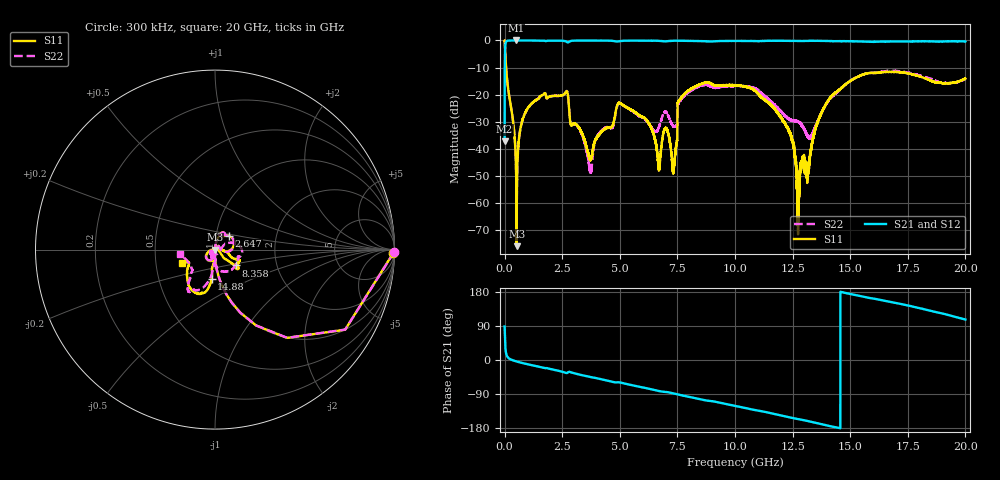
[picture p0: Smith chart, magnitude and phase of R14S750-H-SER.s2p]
!{R14S750}
!Johanson Technology Inc.
!www.johansontechnology.com
!Test Board Conditions:
!Substrate Type  RO4350B
!Substrate Thickness  20 mil
!Substrate Dk  3.66
!TL Type: GCPW
!TL Trace Width  36 mil
!TL Gap  12 mil
!Electrode orientation  Horizontal
!DUT TOPOLOGY	SERIES
!Mounting Pad LxW  26x36 mil
! Created Wed Nov 25 17:33:21 2020
! 2 Port Network Data from SP1.SP block
! freq  magS11  angS11  magS21  angS21  magS12  angS12  magS22  angS22
# khz S ma R 50
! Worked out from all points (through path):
!   20001 points, 300 kHz to 20 GHz, reference 50 ohm
!   highest |S21| = 0.00 dB at 498.3 MHz (marker M1); lowest = -37.2 dB at 300 kHz (marker M2)
!   group delay of S21, straight-line fit = 35 ps
!   lowest |S11| = -75.9 dB at 524.3 MHz (marker M3), VSWR 1.00, Z = 50 - j0.00839 ohm
!   |S11| at or under -10 dB: 64.05 MHz to end of sweep
!   |S22| runs from -70.4 to 0.0 dB; largest |S21 - S12| = 0.017
!   S11 on the Smith chart (normalised r, x): 300 kHz: open; 2.647 GHz: 1.16, +0.18; 8.358 GHz: 1.24, -0.23; 14.88 GHz: 0.91, -0.31; 20 GHz: 0.68, -0.10
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300  0.9937 -1.1  0.01383 88.4  0.01379 89.1  0.9972 -0.9
109300  0.1871 -80.1  0.982 9.9  0.9818 9.9  0.1877 -80.1
498300  0.004191 -92.3  1 -3.6  0.9994 -3.5  0.004227 -95.8
524300  0.0001607 -31.4  0.9993 -4.0  0.9998 -4.0  0.0003109 -154.3
1047300  0.05956 77.4  0.9975 -11.8  0.9976 -11.8  0.05937 78.6
2647300  0.1099 43.8  0.9671 -33.8  0.9674 -33.8  0.1104 42.2
3334300  0.02031 44.5  0.9958 -39.6  0.9965 -39.7  0.0194 41.0
3729300  0.006442 -10.8  0.9934 -45.0  0.9941 -45.0  0.003877 -12.6
5030300  0.0693 -130.6  0.9749 -59.6  0.9745 -59.6  0.06833 -133.7
6226300  0.03073 -168.8  0.9908 -75.3  0.9912 -75.4  0.03037 -142.0
6667300  0.005541 -157.4  0.985 -81.5  0.9846 -81.5  0.02331 -86.2
6999300  0.02413 -114.1  0.9639 -84.4  0.9636 -84.4  0.04792 -95.4
7344300  0.00448 80.8  0.9866 -88.4  0.9881 -88.4  0.02557 -82.8
7600300  0.0806 -41.3  0.9873 -92.0  0.9876 -91.9  0.07508 28.3
8358300  0.1472 -37.0  0.9787 -101.8  0.978 -101.8  0.1378 8.7
1.00003e7  0.1497 -23.8  0.98 -121.1  0.98 -121.1  0.1449 -43.1
1.22063e7  0.02737 3.6  0.9855 -149.2  0.9876 -149.1  0.0389 -123.2
1.27423e7  0.0004717 155.2  0.9756 -156.0  0.9773 -156.1  0.03211 -150.5
1.33343e7  0.01168 -98.9  0.9844 -163.5  0.9853 -163.5  0.01789 -115.8
1.48793e7  0.1649 -96.6  0.9693 175.8  0.9692 175.6  0.1656 -99.8
1.66673e7  0.2612 -111.9  0.9572 154.2  0.9496 154.0  0.276 -120.9
2e7  0.1984 -158.3  0.9596 106.7  0.9592 106.9  0.1961 -172.9
